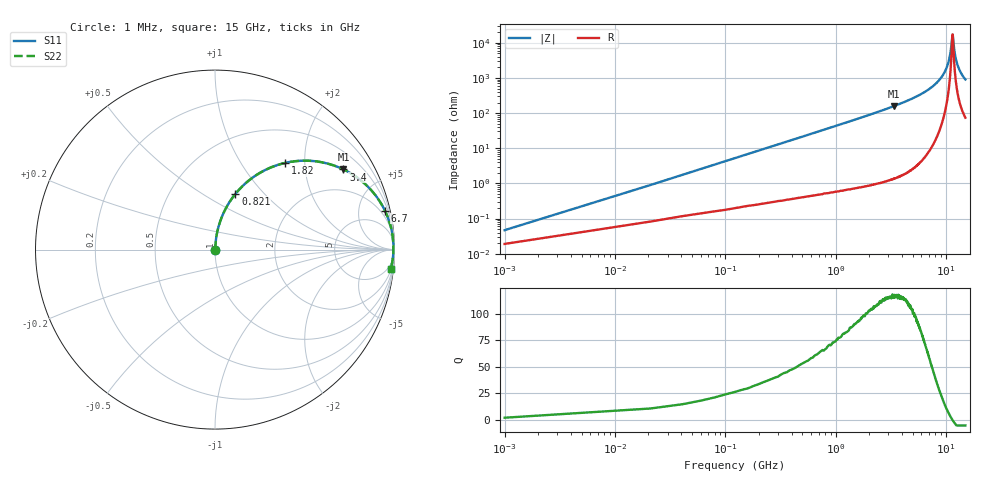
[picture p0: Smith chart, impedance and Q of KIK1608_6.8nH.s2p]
!version-2
!date-01.2022
!Series
# MHz S RI R 50
!Freq ReS11 ImS11 ReS21 ImS21 ReS12 ImS12 ReS22 ImS22
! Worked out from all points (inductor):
!   751 points, 1 MHz to 15 GHz, reference 50 ohm
!   read as one part in series: L = 6.8 nH near 61 MHz
!   highest Q = 117 at 3.4 GHz (marker M1), where L = 7.46 nH
!   self-resonance near 11.48 GHz
!   S11 on the Smith chart (normalised r, x): 1 MHz: 1.00, +0.00; 821 MHz: 1.01, +0.71; 1.82 GHz: 1.02, +1.60; 3.4 GHz: 1.03, +3.19; 6.7 GHz: 1.13, +8.69; 15 GHz: 2, -18
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1  0.00018 0.000427  0.9998 -0.000427  0.9998 -0.000427  0.00018 0.000427
81  0.0028 0.0345  0.9972 -0.0345  0.9972 -0.0345  0.0028 0.0345
121  0.00462 0.0514  0.9954 -0.0514  0.9954 -0.0514  0.00462 0.0514
181  0.00831 0.0765  0.9917 -0.0765  0.9917 -0.0765  0.00831 0.0765
281  0.0171 0.1177  0.9829 -0.1177  0.9829 -0.1177  0.0171 0.1177
421  0.0348 0.1732  0.9652 -0.1732  0.9652 -0.1732  0.0348 0.1732
821  0.1142 0.3107  0.8858 -0.3107  0.8858 -0.3107  0.1142 0.3107
1260  0.232 0.4161  0.768 -0.4161  0.768 -0.4161  0.232 0.4161
1820  0.3902 0.4827  0.6098 -0.4827  0.6098 -0.4827  0.3902 0.4827
2520  0.561 0.4918  0.439 -0.4918  0.439 -0.4918  0.561 0.4918
3400  0.7156 0.4468  0.2844 -0.4468  0.2844 -0.4468  0.7156 0.4468
5020  0.8731 0.3279  0.1269 -0.3279  0.1269 -0.3279  0.8731 0.3279
6700  0.9467 0.2172  0.0533 -0.2172  0.0533 -0.2172  0.9467 0.2172
7520  0.9661 0.171  0.0339 -0.171  0.0339 -0.171  0.9661 0.171
8980  0.9858 0.0993  0.0142 -0.0993  0.0142 -0.0993  0.9858 0.0993
10020  0.9922 0.0549  0.0078 -0.0549  0.0078 -0.0549  0.9922 0.0549
10840  0.9942 0.0232  0.00583 -0.0232  0.00583 -0.0232  0.9942 0.0232
11480  0.9942 4.1e-05  0.00575 -4.1e-05  0.00575 -4.1e-05  0.9942 4.1e-05
12000  0.9935 -0.0178  0.00648 0.0178  0.00648 0.0178  0.9935 -0.0178
12520  0.9922 -0.0348  0.00781 0.0348  0.00781 0.0348  0.9922 -0.0348
13520  0.9882 -0.0656  0.0118 0.0656  0.0118 0.0656  0.9882 -0.0656
15000  0.9794 -0.1069  0.0206 0.1069  0.0206 0.1069  0.9794 -0.1069
